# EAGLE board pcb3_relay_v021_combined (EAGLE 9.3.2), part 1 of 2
2022-05-20: PCB made by JLCPCB
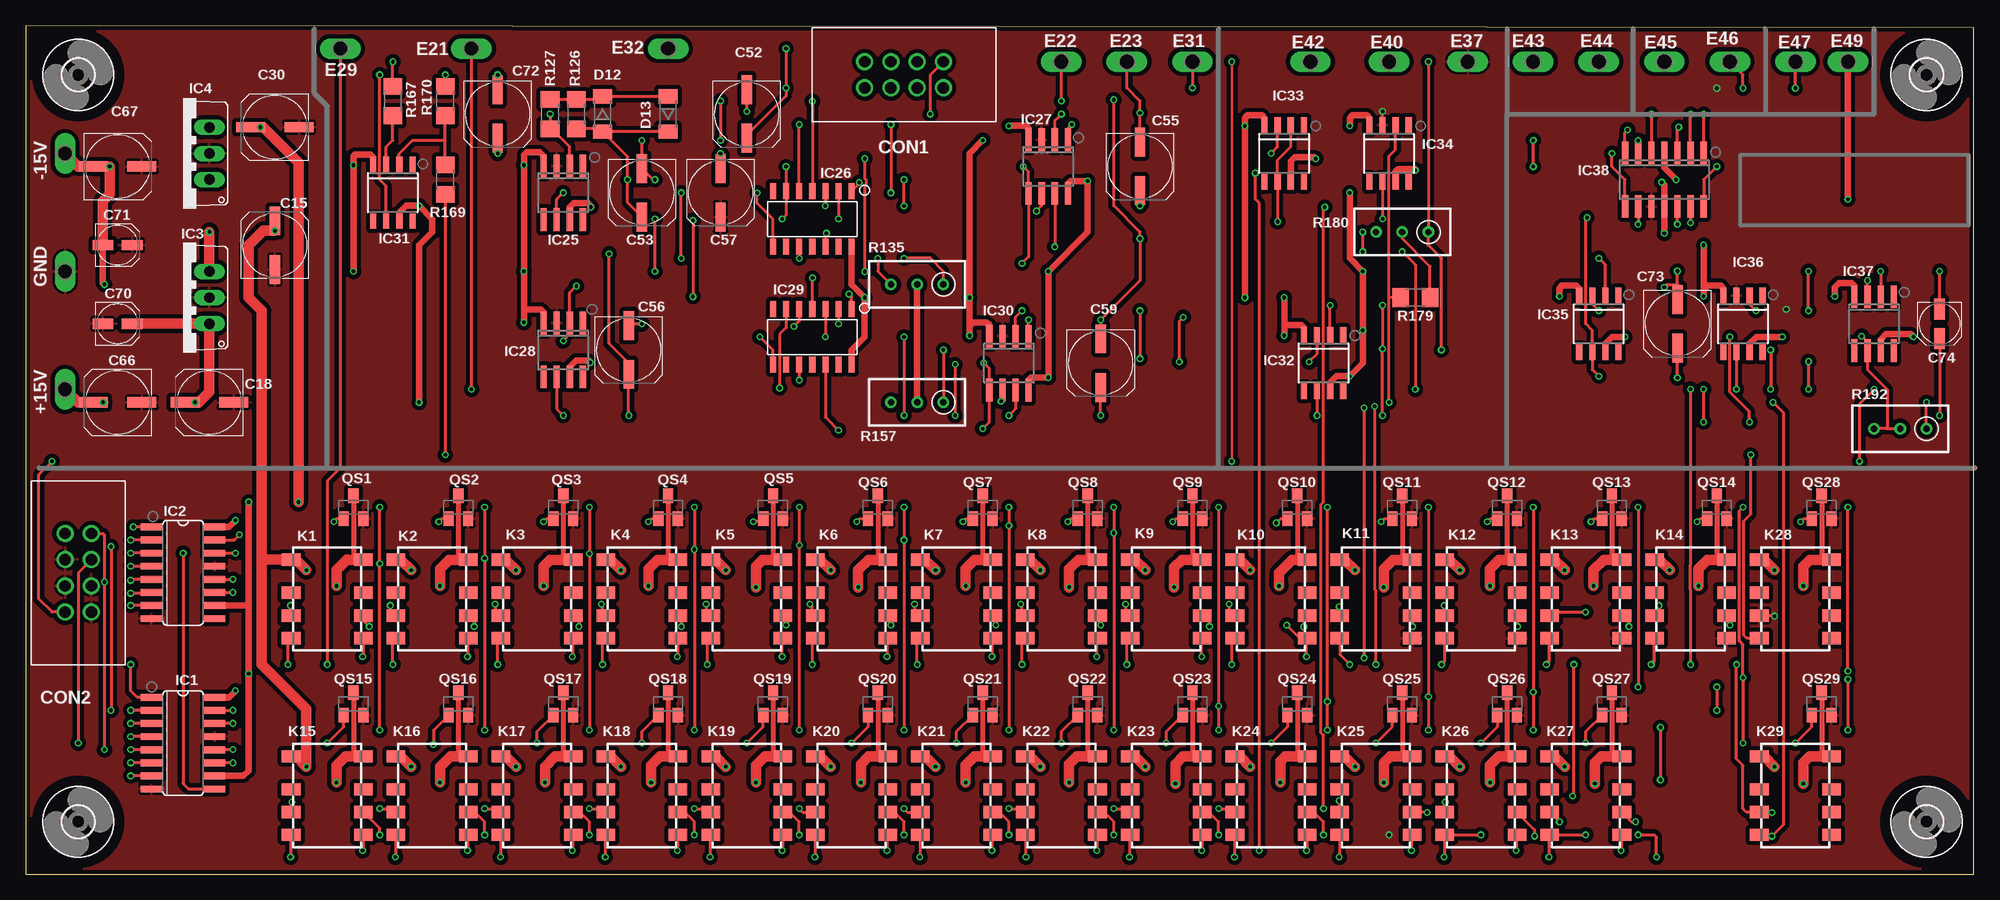
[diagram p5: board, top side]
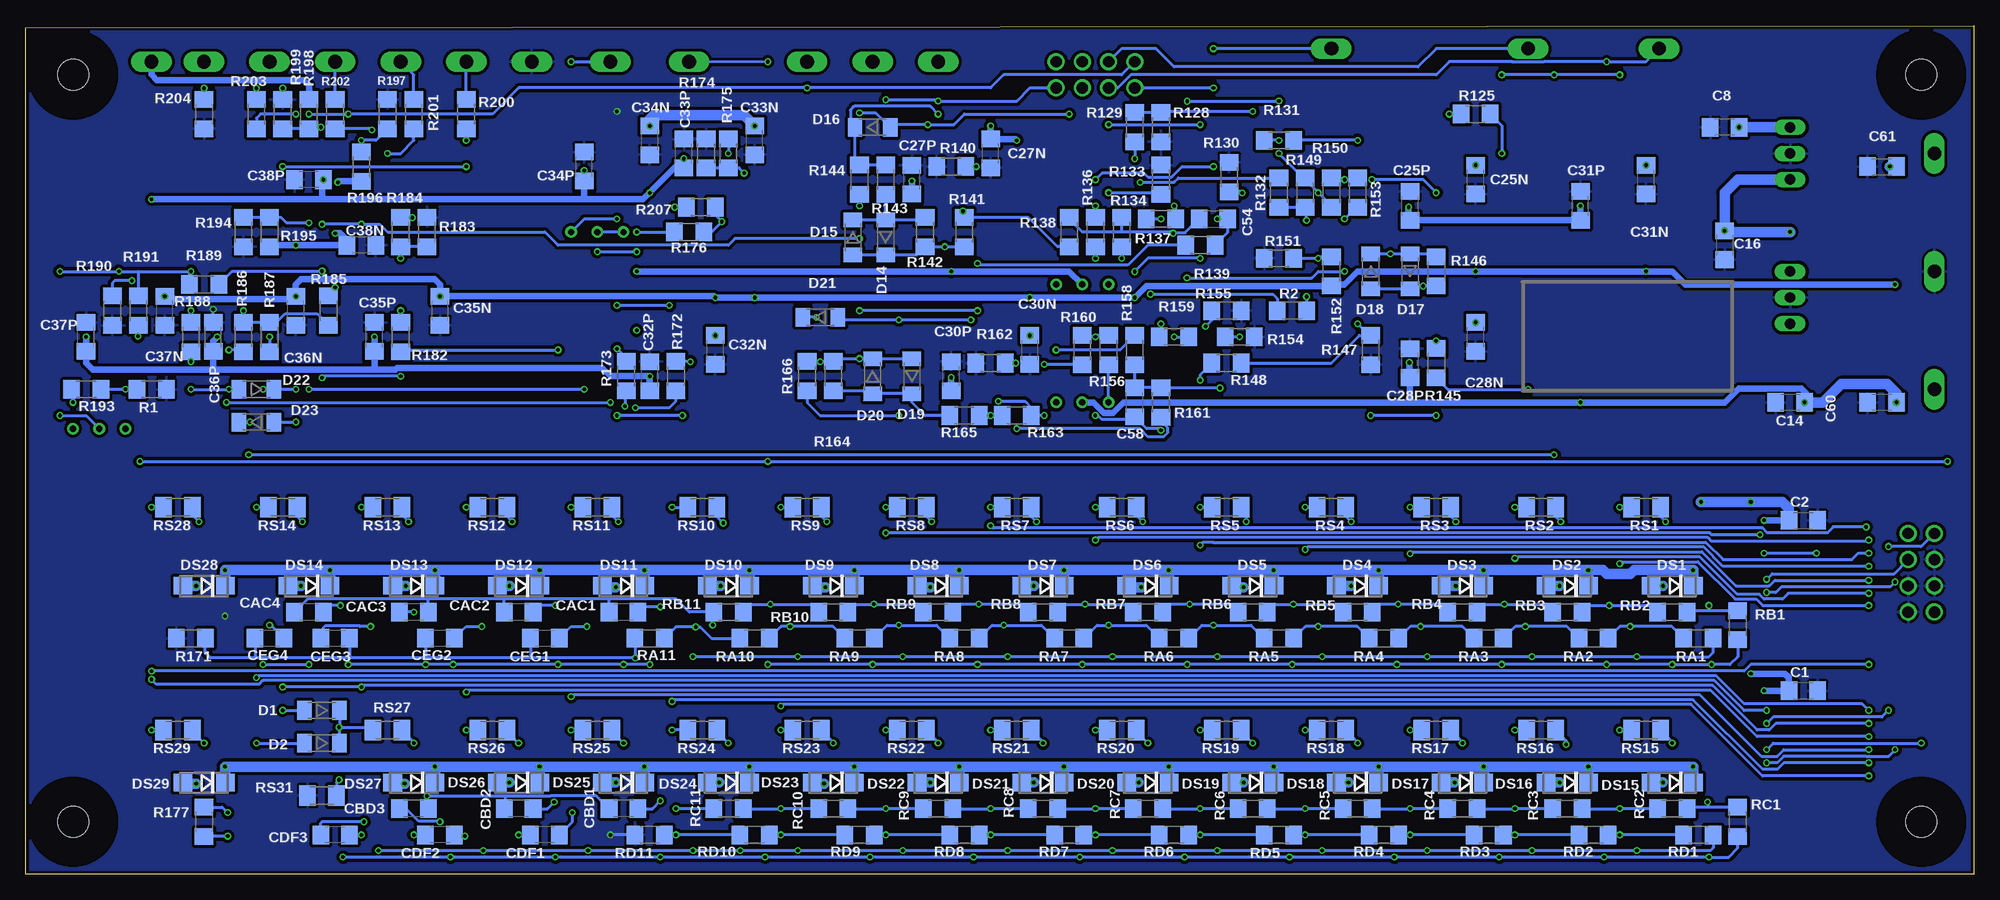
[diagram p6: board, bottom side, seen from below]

Size 188.72 x 82.22 mm. Coordinates in mm from the lower left corner, seen from the top.
Outline: 0,0 188.72,0 188.72,82.04 0,82.22 0,0
Copper layers (1*16): Top 0.035mm / dielectric 1.5mm / Bottom 0.035mm
Design rules "ITEADstudio_DRC for Eagle v6": minimum track width 6mil, minimum drill 12mil, track to track 6mil, track to pad 6mil, pad to pad 6mil, via to via 6mil, smd to smd 0mil, copper to edge 10mil, drill to drill 10mil, minimum pad ring 10mil, minimum via ring 6mil, stop-mask expansion 2mil, vias tented up to drill 100mil, thermal gap 10mil

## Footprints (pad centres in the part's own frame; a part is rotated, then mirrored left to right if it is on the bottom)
P1-13Y = drill 1.321 pad 1.905 long: TP 0,0
C1206 = smd 1.6 x 1.8: 1 -1.4,0; 2 1.4,0
UD-6,3X5,8_NICHICON = smd 2.8 x 1: + 2.35,0; - -2.35,0
UD-4X5,8_NICHICON = smd 2 x 1: + 1.425,0; - -1.425,0
61200821621 = drill 1.1: 1 -2.54,-1.27; 2 -2.54,1.27; 3 0,-1.27; 4 0,1.27; 5 2.54,-1.27; 6 2.54,1.27; 7 5.08,-1.27; 8 5.08,1.27
SOD80 = smd 1.4 x 1.8: 1 -1.7,0; 2 1.7,0
DO214AC = smd 1.8 x 1.7: A 2.05,0; C -2.05,0
SO16 = smd 0.66 x 2.032: 1 -4.445,-3.073; 2 -3.175,-3.073; 3 -1.905,-3.073; 4 -0.635,-3.073; 5 0.635,-3.073; 6 1.905,-3.073; 7 3.175,-3.073; 8 4.445,-3.073; 9 4.445,3.073; 10 3.175,3.073; 11 1.905,3.073; 12 0.635,3.073; 13 -0.635,3.073; 14 -1.905,3.073; 15 -3.175,3.073; 16 -4.445,3.073
TO220V = drill 1.016 long: 1 -2.54,-2.54; 2 0,-2.54; 3 2.54,-2.54
SO08 = smd 0.6 x 2.2: 1 -1.905,-2.6; 2 -0.635,-2.6; 3 0.635,-2.6; 4 1.905,-2.6; 5 1.905,2.6; 6 0.635,2.6; 7 -0.635,2.6; 8 -1.905,2.6
SOIC-14 = smd 0.6 x 1.55: 1 -3.81,-2.7; 2 -2.54,-2.7; 3 -1.27,-2.7; 4 0,-2.7; 5 1.27,-2.7; 6 2.54,-2.7; 7 3.81,-2.7; 8 3.81,2.7; 9 2.54,2.7; 10 1.27,2.7; 11 0,2.7; 12 -1.27,2.7; 13 -2.54,2.7; 14 -3.81,2.7
SOIC8 = smd 0.6 x 1.5: 1 -1.905,-2.75; 2 -0.635,-2.75; 3 0.635,-2.75; 4 1.905,-2.75; 5 1.905,2.75; 6 0.635,2.75; 7 -0.635,2.75; 8 -1.905,2.75
SO14 = smd 0.6 x 2.2: 1 -3.81,-2.6; 2 -2.54,-2.6; 3 -1.27,-2.6; 4 0,-2.6; 5 1.27,-2.6; 6 2.54,-2.6; 7 3.81,-2.6; 8 3.81,2.6; 9 2.54,2.6; 10 1.27,2.6; 11 0,2.6; 12 -1.27,2.6; 13 -2.54,2.6; 14 -3.81,2.6
G6K-2F-Y = smd 1.2 x 1.8: 1 -3.8,-3.5; 2 -0.6,-3.5; 3 1.6,-3.5; 4 3.8,-3.5; 5 3.8,3.5; 6 1.6,3.5; 7 -0.6,3.5; 8 -3.8,3.5
SOT23 = smd 1 x 1.4: 1 -0.95,-1.1; 2 0.95,-1.1; 3 0,1.1
R1206 = smd 1.6 x 1.803: 1 -1.422,0; 2 1.422,0
RTRIM3296W = drill 0.61: 1 0,-2.54; 2 0,0; 3 0,2.54
M1206 = smd 1.6 x 2: 1 -1.4,0; 2 1.4,0
3,0 = hole 3: 0,0

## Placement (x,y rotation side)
+15V  TPPAD1-13Y  [P1-13Y]  3.81,46.99 0 top
-15V  TPPAD1-13Y  [P1-13Y]  3.81,69.85 0 top
C1  100n  [C1206]  16.51,17.78 0 bottom
C2  100n  [C1206]  16.51,34.29 0 bottom
C8  100n  [C1206]  24.13,72.39 180 bottom
C14  100n  [C1206]  17.78,45.72 180 bottom
C15  100u/16V  [UD-6,3X5,8_NICHICON]  24.13,60.96 90 top
C16  100n  [C1206]  24.13,60.96 270 bottom
C18  100u/16V  [UD-6,3X5,8_NICHICON]  17.78,45.72 180 top
C25N  100n  [C1206]  48.26,67.31 90 bottom
C25P  100n  [C1206]  54.61,64.77 90 bottom
C27N  100n  [C1206]  95.25,69.85 90 bottom
C27P  100n  [C1206]  102.87,67.31 90 bottom
C28N  100n  [C1206]  48.26,52.07 90 bottom
C28P  100n  [C1206]  54.61,49.53 90 bottom
C30  100u/16V  [UD-6,3X5,8_NICHICON]  24.13,72.39 180 top
C30N  100n  [C1206]  91.44,50.8 90 bottom
C30P  100n  [C1206]  99.06,48.26 90 bottom
C31N  100n  [C1206]  31.75,67.31 90 bottom
C31P  100n  [C1206]  38.1,64.77 90 bottom
C32N  100n  [C1206]  121.92,50.8 90 bottom
C32P  100n  [C1206]  128.27,48.26 90 bottom
C33N  100n  [C1206]  118.11,71.12 90 bottom
C33P  100n  [C1206]  124.97,69.85 90 bottom
C34N  100n  [C1206]  128.27,71.12 90 bottom
C34P  100n  [C1206]  134.62,68.58 90 bottom
C35N  100n  [C1206]  148.59,54.61 90 bottom
C35P  100n  [C1206]  154.94,52.07 90 bottom
C36N  100n  [C1206]  162.56,54.61 90 bottom
C36P  100n  [C1206]  170.56,52.07 90 bottom
C37N  100n  [C1206]  175.26,54.61 90 bottom
C37P  100n  [C1206]  182.88,52.07 90 bottom
C38N  100n  [C1206]  156.21,60.96 180 bottom
C38P  100n  [C1206]  161.29,67.31 180 bottom
C52  100u/16V  [UD-6,3X5,8_NICHICON]  69.85,73.66 270 top
C53  100u/16V  [UD-6,3X5,8_NICHICON]  59.69,66.04 270 top
C54  0.47uF  [C1206]  73.66,63.5 0 bottom
C55  100u/16V  [UD-6,3X5,8_NICHICON]  107.95,68.58 270 top
C56  100u/16V  [UD-6,3X5,8_NICHICON]  58.42,50.8 270 top
C57  100u/16V  [UD-6,3X5,8_NICHICON]  67.31,66.04 270 top
C58  0.47uF  [C1206]  81.28,45.72 90 bottom
C59  100u/16V  [UD-6,3X5,8_NICHICON]  104.14,49.53 270 top
C60  100n  [C1206]  8.89,45.72 180 bottom
C61  100n  [C1206]  8.89,68.58 0 bottom
C66  100u/16V  [UD-6,3X5,8_NICHICON]  8.89,45.72 180 top
C67  100u/16V  [UD-6,3X5,8_NICHICON]  8.89,68.58 0 top
C70  1u/50V  [UD-4X5,8_NICHICON]  8.89,53.34 0 top
C71  1u/50V  [UD-4X5,8_NICHICON]  8.89,60.96 0 top
C72  100u/16V  [UD-6,3X5,8_NICHICON]  45.72,73.66 270 top
C73  100u/16V  [UD-6,3X5,8_NICHICON]  160.02,53.34 270 top
C74  1u/50V  [UD-4X5,8_NICHICON]  185.42,53.34 270 top
CAC1  100n  [C1206]  130.81,25.4 180 bottom
CAC2  10n  [C1206]  140.97,25.4 180 bottom
CAC3  1n  [C1206]  151.13,25.4 180 bottom
CAC4  100p  [C1206]  161.29,25.4 180 bottom
CBD1  220n  [C1206]  130.81,6.35 180 bottom
CBD2  22n  [C1206]  140.97,6.35 180 bottom
CBD3  2n2  [C1206]  151.13,6.35 180 bottom
CDF1  220n  [C1206]  138.43,3.81 180 bottom
CDF2  22n  [C1206]  148.59,3.81 180 bottom
CDF3  2n2  [C1206]  158.75,3.81 180 bottom
CEG1  68n  [C1206]  138.43,22.86 180 bottom
CEG2  6n8  [C1206]  148.59,22.86 180 bottom
CEG3  680p  [C1206]  158.75,22.86 180 bottom
CEG4  47p  [C1206]  165.1,22.86 180 bottom
CON1  PCB2_IO  [61200821621]  83.82,77.47 0 top
CON2  UC_IO  [61200821621]  5.08,27.94 90 top
D1  1N4148  [SOD80]  160.02,15.88 180 bottom
D2  1N4148  [SOD80]  160.02,12.7 180 bottom
D12  1N4148  [SOD80]  55.88,73.66 270 top
D13  1N4148  [SOD80]  62.23,73.66 90 top
D14  1N4148  [SOD80]  105.41,61.72 90 bottom
D15  1N4148  [SOD80]  108.58,61.72 270 bottom
D16  1N4148  [SOD80]  106.68,72.39 0 bottom
D17  1N4148  [SOD80]  54.61,58.42 90 bottom
D18  1N4148  [SOD80]  58.42,58.42 270 bottom
D19  1N4148  [SOD80]  102.87,48.26 90 bottom
D20  1N4148  [SOD80]  106.68,48.26 270 bottom
D21  1N4148  [SOD80]  111.76,53.98 0 bottom
D22  1N4148  [SOD80]  166.37,46.99 180 bottom
D23  1N4148  [SOD80]  166.37,43.81 0 bottom
DS1  M7  [DO214AC]  29.21,27.94 180 bottom
DS2  M7  [DO214AC]  39.37,27.94 180 bottom
DS3  M7  [DO214AC]  49.53,27.94 180 bottom
DS4  M7  [DO214AC]  59.69,27.94 180 bottom
DS5  M7  [DO214AC]  69.85,27.94 180 bottom
DS6  M7  [DO214AC]  80.01,27.94 180 bottom
DS7  M7  [DO214AC]  90.17,27.94 180 bottom
DS8  M7  [DO214AC]  100.33,27.94 180 bottom
DS9  M7  [DO214AC]  110.49,27.94 180 bottom
DS10  M7  [DO214AC]  120.65,27.94 180 bottom
DS11  M7  [DO214AC]  130.81,27.94 180 bottom
DS12  M7  [DO214AC]  140.97,27.94 180 bottom
DS13  M7  [DO214AC]  151.13,27.94 180 bottom
DS14  M7  [DO214AC]  161.29,27.94 180 bottom
DS15  M7  [DO214AC]  29.21,8.89 180 bottom
DS16  M7  [DO214AC]  39.37,8.89 180 bottom
DS17  M7  [DO214AC]  49.53,8.89 180 bottom
DS18  M7  [DO214AC]  59.69,8.89 180 bottom
DS19  M7  [DO214AC]  69.85,8.89 180 bottom
DS20  M7  [DO214AC]  80.01,8.89 180 bottom
DS21  M7  [DO214AC]  90.17,8.89 180 bottom
DS22  M7  [DO214AC]  100.33,8.89 180 bottom
DS23  M7  [DO214AC]  110.49,8.89 180 bottom
DS24  M7  [DO214AC]  120.65,8.89 180 bottom
DS25  M7  [DO214AC]  130.81,8.89 180 bottom
DS26  M7  [DO214AC]  140.97,8.89 180 bottom
DS27  M7  [DO214AC]  151.13,8.89 180 bottom
DS28  M7  [DO214AC]  171.45,27.94 180 bottom
DS29  M7  [DO214AC]  171.45,8.89 180 bottom
E21  TPPAD1-13Y  [P1-13Y]  43.18,80.01 90 top
E22  TPPAD1-13Y  [P1-13Y]  100.33,78.74 90 top
E23  TPPAD1-13Y  [P1-13Y]  106.68,78.74 90 top
E29  TPPAD1-13Y  [P1-13Y]  30.48,80.01 270 top
E31  TPPAD1-13Y  [P1-13Y]  113.03,78.74 90 top
E32  TPPAD1-13Y  [P1-13Y]  62.23,80.01 90 top
E37  TPPAD1-13Y  [P1-13Y]  139.7,78.74 90 top
E40  TPPAD1-13Y  [P1-13Y]  132.08,78.74 90 top
E42  TPPAD1-13Y  [P1-13Y]  124.46,78.74 90 top
E43  TPPAD1-13Y  [P1-13Y]  146.05,78.74 90 top
E44  TPPAD1-13Y  [P1-13Y]  152.4,78.74 90 top
E45  TPPAD1-13Y  [P1-13Y]  158.75,78.74 90 top
E46  TPPAD1-13Y  [P1-13Y]  165.1,78.74 90 top
E47  TPPAD1-13Y  [P1-13Y]  171.45,78.74 90 top
E49  TPPAD1-13Y  [P1-13Y]  176.53,78.74 90 top
GND  TPPAD1-13Y  [P1-13Y]  3.81,58.42 0 top
IC1  74HC595D  [SO16]  15.24,12.7 270 top
IC2  74HC595D  [SO16]  15.24,29.21 270 top
IC3  7812TV  [TO220V]  15.24,55.88 90 top
IC4  7805TV  [TO220V]  15.24,69.85 90 top
IC25  LM318D  [SO08]  52.07,66.04 180 top
IC26  MC1496D  [SOIC-14]  76.2,63.5 180 top
IC27  LM1458D  [SO08]  99.06,68.58 180 top
IC28  LM318D  [SO08]  52.07,50.8 180 top
IC29  MC1496D  [SOIC-14]  76.2,52.07 180 top
IC30  LM1458D  [SO08]  95.25,49.53 180 top
IC31  LM318D  [SOIC8]  35.56,66.04 180 top
IC32  LM318D  [SOIC8]  125.73,49.53 180 top
IC33  LM318D  [SOIC8]  121.92,69.85 180 top
IC34  LM318D  [SOIC8]  132.08,69.85 180 top
IC35  LM318D  [SOIC8]  152.4,53.34 180 top
IC36  LM318D  [SOIC8]  166.37,53.34 180 top
IC37  LM741D  [SO08]  179.07,53.34 180 top
IC38  LM324D  [SO14]  158.75,67.31 180 top
K1  G6K-2F-Y  [G6K-2F-Y]  29.21,26.67 270 top
K2  G6K-2F-Y  [G6K-2F-Y]  39.37,26.67 270 top
K3  G6K-2F-Y  [G6K-2F-Y]  49.53,26.67 270 top
K4  G6K-2F-Y  [G6K-2F-Y]  59.69,26.67 270 top
K5  G6K-2F-Y  [G6K-2F-Y]  69.85,26.67 270 top
K6  G6K-2F-Y  [G6K-2F-Y]  80.01,26.67 270 top
K7  G6K-2F-Y  [G6K-2F-Y]  90.17,26.67 270 top
K8  G6K-2F-Y  [G6K-2F-Y]  100.33,26.67 270 top
K9  G6K-2F-Y  [G6K-2F-Y]  110.49,26.67 270 top
K10  G6K-2F-Y  [G6K-2F-Y]  120.65,26.67 270 top
K11  G6K-2F-Y  [G6K-2F-Y]  130.81,26.67 270 top
K12  G6K-2F-Y  [G6K-2F-Y]  140.97,26.67 270 top
K13  G6K-2F-Y  [G6K-2F-Y]  151.13,26.67 270 top
K14  G6K-2F-Y  [G6K-2F-Y]  161.29,26.67 270 top
K15  G6K-2F-Y  [G6K-2F-Y]  29.21,7.62 270 top
K16  G6K-2F-Y  [G6K-2F-Y]  39.37,7.62 270 top
K17  G6K-2F-Y  [G6K-2F-Y]  49.53,7.62 270 top
K18  G6K-2F-Y  [G6K-2F-Y]  59.69,7.62 270 top
K19  G6K-2F-Y  [G6K-2F-Y]  69.85,7.62 270 top
K20  G6K-2F-Y  [G6K-2F-Y]  80.01,7.62 270 top
K21  G6K-2F-Y  [G6K-2F-Y]  90.17,7.62 270 top
K22  G6K-2F-Y  [G6K-2F-Y]  100.33,7.62 270 top
K23  G6K-2F-Y  [G6K-2F-Y]  110.49,7.62 270 top
K24  G6K-2F-Y  [G6K-2F-Y]  120.65,7.62 270 top
K25  G6K-2F-Y  [G6K-2F-Y]  130.81,7.62 270 top
K26  G6K-2F-Y  [G6K-2F-Y]  140.97,7.62 270 top
K27  G6K-2F-Y  [G6K-2F-Y]  151.13,7.62 270 top
K28  G6K-2F-Y  [G6K-2F-Y]  171.45,26.67 270 top
K29  G6K-2F-Y  [G6K-2F-Y]  171.45,7.62 270 top
QS1  SS8050  [SOT23]  31.75,35.56 0 top
QS2  SS8050  [SOT23]  41.91,35.56 0 top
QS3  SS8050  [SOT23]  52.07,35.56 0 top
QS4  SS8050  [SOT23]  62.23,35.56 0 top
QS5  SS8050  [SOT23]  72.39,35.56 0 top
QS6  SS8050  [SOT23]  82.55,35.56 0 top
QS7  SS8050  [SOT23]  92.71,35.56 0 top
QS8  SS8050  [SOT23]  102.87,35.56 0 top
QS9  SS8050  [SOT23]  113.03,35.56 0 top
QS10  SS8050  [SOT23]  123.19,35.56 0 top
QS11  SS8050  [SOT23]  133.35,35.56 0 top
QS12  SS8050  [SOT23]  143.51,35.56 0 top
QS13  SS8050  [SOT23]  153.67,35.56 0 top
QS14  SS8050  [SOT23]  163.83,35.56 0 top
QS15  SS8050  [SOT23]  31.75,16.51 0 top
QS16  SS8050  [SOT23]  41.91,16.51 0 top
QS17  SS8050  [SOT23]  52.07,16.51 0 top
QS18  SS8050  [SOT23]  62.23,16.51 0 top
QS19  SS8050  [SOT23]  72.39,16.51 0 top
QS20  SS8050  [SOT23]  82.55,16.51 0 top
QS21  SS8050  [SOT23]  92.71,16.51 0 top
QS22  SS8050  [SOT23]  102.87,16.51 0 top
QS23  SS8050  [SOT23]  113.03,16.51 0 top
QS24  SS8050  [SOT23]  123.19,16.51 0 top
QS25  SS8050  [SOT23]  133.35,16.51 0 top
QS26  SS8050  [SOT23]  143.51,16.51 0 top
QS27  SS8050  [SOT23]  153.67,16.51 0 top
QS28  SS8050  [SOT23]  173.99,35.56 0 top
QS29  SS8050  [SOT23]  173.99,16.51 0 top
R1  3K3  [R1206]  176.53,46.99 180 bottom
R2  100  [R1206]  66.04,54.61 180 bottom
R125  4K7  [R1206]  48.26,73.66 0 bottom
R126  22k  [R1206]  53.34,73.66 270 top
R127  2K7  [R1206]  50.8,73.66 90 top
R128  1K  [R1206]  78.74,72.39 270 bottom
R129  100  [R1206]  81.28,72.39 90 bottom
R130  100  [R1206]  72.14,67.56 90 bottom
R131  100  [R1206]  67.31,71.12 0 bottom
R132  100  [R1206]  67.31,66.04 270 bottom
R133  22k  [R1206]  78.74,67.31 90 bottom
R134  10k  [R1206]  82.55,62.23 90 bottom
R135  1k  [RTRIM3296W]  86.36,57.15 90 top
R136  10k  [R1206]  85.09,62.23 270 bottom
R137  1K5  [R1206]  78.74,63.5 0 bottom
R138  22k  [R1206]  87.63,62.23 90 bottom
R139  22k  [R1206]  74.93,60.96 180 bottom
R140  6K8  [R1206]  99.06,68.58 180 bottom
R141  6K8  [R1206]  97.79,62.23 90 bottom
R142  100k  [R1206]  101.6,62.23 270 bottom
R143  10k  [R1206]  105.41,67.31 270 bottom
R144  68  [R1206]  107.95,67.31 90 bottom
R145  10k  [R1206]  52.07,49.53 270 bottom
R146  100k  [R1206]  52.07,58.42 90 bottom
R147  10k  [R1206]  58.42,50.8 270 bottom
R148  100  [R1206]  72.39,49.53 0 bottom
R149  1K  [R1206]  64.77,66.04 270 bottom
R150  1K  [R1206]  62.23,66.04 90 bottom
R151  4K7  [R1206]  67.31,59.69 0 bottom
R152  4K7  [R1206]  62.23,58.42 90 bottom
R153  100  [R1206]  59.69,66.04 270 bottom
R154  100  [R1206]  71.12,52.07 0 bottom
R155  22k  [R1206]  72.39,54.61 0 bottom
R156  10k  [R1206]  83.82,50.8 90 bottom
R157  1k  [RTRIM3296W]  86.36,45.72 90 top
R158  10k  [R1206]  81.28,50.8 90 bottom
R159  1K5  [R1206]  77.47,52.07 0 bottom
R160  22k  [R1206]  86.36,50.8 90 bottom
R161  22k  [R1206]  78.74,45.72 270 bottom
R162  6K8  [R1206]  95.25,49.53 180 bottom
R163  6K8  [R1206]  92.71,44.45 0 bottom
R164  100k  [R1206]  110.49,48.26 270 bottom
R165  10k  [R1206]  97.79,44.45 0 bottom
R166  68  [R1206]  113.03,48.26 90 bottom
R167  100  [R1206]  35.56,74.93 270 top
R169  390  [R1206]  40.64,67.31 270 top
R170  3K3  [R1206]  40.64,74.93 270 top
R171  100k  [R1206]  172.72,22.86 0 bottom
R172  100  [R1206]  125.73,48.26 90 bottom
R173  100  [R1206]  130.56,48.26 270 bottom
R174  100k  [R1206]  122.81,69.85 270 bottom
R175  100  [R1206]  120.65,69.85 90 bottom
R176  1K  [R1206]  124.46,62.23 180 bottom
R177  9k09  [R1206]  171.45,5.08 270 bottom
R179  3K  [R1206]  134.62,55.88 0 top
R180  2K  [RTRIM3296W]  133.35,62.23 90 top
R182  100  [R1206]  152.4,52.07 90 bottom
R183  1K  [R1206]  149.86,62.23 90 bottom
R184  9K1  [R1206]  152.4,62.23 270 bottom
R185  1K  [R1206]  159.38,54.61 90 bottom
R186  1K  [R1206]  167.64,52.07 270 bottom
R187  1K  [R1206]  165.1,52.07 90 bottom
R188  10k  [R1206]  172.72,52.07 90 bottom
R189  20k  [R1206]  171.45,57.15 0 bottom
R190  6K8  [R1206]  180.34,54.61 90 bottom
R191  270k  [R1206]  177.8,54.61 270 bottom
R192  5k  [RTRIM3296W]  181.61,43.18 90 top
R193  4K7  [R1206]  182.88,46.99 180 bottom
R194  39k  [R1206]  167.64,62.23 90 bottom
R195  10k  [R1206]  165.1,62.23 90 bottom
R196  33k  [R1206]  156.21,68.58 90 bottom
R197  10k  [R1206]  153.67,73.66 270 bottom
R198  33k  [R1206]  161.29,73.66 270 bottom
R199  10k  [R1206]  163.83,73.66 270 bottom
R200  2K7  [R1206]  146.05,73.66 90 bottom
R201  2K7  [R1206]  151.13,73.66 90 bottom
R202  2K7  [R1206]  158.75,73.66 90 bottom
R203  2K7  [R1206]  166.37,73.66 90 bottom
R204  1K5  [R1206]  171.45,73.66 90 bottom
R207  100  [R1206]  123.32,64.64 0 bottom
RA1  1K5  [R1206]  26.67,22.86 180 bottom
RA2  1K  [R1206]  36.83,22.86 180 bottom
RA3  1K3  [R1206]  46.99,22.86 180 bottom
RA4  750  [R1206]  57.15,22.86 180 bottom
RA5  680  [R1206]  67.31,22.86 180 bottom
RA6  430  [R1206]  77.47,22.86 180 bottom
RA7  360  [R1206]  87.63,22.86 180 bottom
RA8  330  [R1206]  97.79,22.86 180 bottom
RA9  220  [R1206]  107.95,22.86 180 bottom
RA10  180  [R1206]  118.11,22.86 180 bottom
RA11  750  [R1206]  128.27,22.86 180 bottom
RB1  1K5  [R1206]  22.86,24.13 90 bottom
RB2  1K  [R1206]  29.21,25.4 180 bottom
RB3  1K3  [R1206]  39.37,25.4 180 bottom
RB4  750  [R1206]  49.53,25.4 180 bottom
RB5  680  [R1206]  59.69,25.4 180 bottom
RB6  430  [R1206]  69.85,25.4 180 bottom
RB7  360  [R1206]  80.01,25.4 180 bottom
RB8  330  [R1206]  90.17,25.4 180 bottom
RB9  220  [R1206]  100.33,25.4 180 bottom
RB10  180  [R1206]  110.49,25.4 180 bottom
RB11  750  [R1206]  120.65,25.4 180 bottom
RC1  3K6  [R1206]  22.86,5.08 90 bottom
RC2  2K4  [R1206]  29.21,6.35 180 bottom
RC3  3K  [R1206]  39.37,6.35 180 bottom
RC4  1K8  [R1206]  49.53,6.35 180 bottom
RC5  1K6  [R1206]  59.69,6.35 180 bottom
RC6  1K  [R1206]  69.85,6.35 180 bottom
RC7  910  [R1206]  80.01,6.35 180 bottom
RC8  820  [R1206]  90.17,6.35 180 bottom
RC9  510  [R1206]  100.33,6.35 180 bottom
RC10  470  [R1206]  110.49,6.35 180 bottom
RC11  1K8  [R1206]  120.65,6.35 180 bottom
RD1  9K1  [R1206]  26.67,3.81 180 bottom
RD2  6K8  [R1206]  36.83,3.81 180 bottom
RD3  7K5  [R1206]  46.99,3.81 180 bottom
RD4  4K7  [R1206]  57.15,3.81 180 bottom
RD5  4K3  [R1206]  67.31,3.81 180 bottom
RD6  2K7  [R1206]  77.47,3.81 180 bottom
RD7  2K4  [R1206]  87.63,3.81 180 bottom
RD8  2K2  [R1206]  97.79,3.81 180 bottom
RD9  1K3  [R1206]  107.95,3.81 180 bottom
RD10  1K2  [R1206]  118.11,3.81 180 bottom
RD11  4K7  [R1206]  128.27,3.81 180 bottom
RS1  4k7  [M1206]  31.75,35.56 180 bottom
RS2  4k7  [M1206]  41.91,35.56 180 bottom
RS3  4k7  [M1206]  52.07,35.56 180 bottom
RS4  4k7  [M1206]  62.23,35.56 180 bottom
RS5  4k7  [M1206]  72.39,35.56 180 bottom
RS6  4k7  [M1206]  82.55,35.56 180 bottom
RS7  4k7  [M1206]  92.71,35.56 180 bottom
RS8  4k7  [M1206]  102.87,35.56 180 bottom
RS9  4k7  [M1206]  113.03,35.56 180 bottom
RS10  4k7  [M1206]  123.19,35.56 180 bottom
RS11  4k7  [M1206]  133.35,35.56 180 bottom
RS12  4k7  [M1206]  143.51,35.56 180 bottom
RS13  4k7  [M1206]  153.67,35.56 180 bottom
RS14  4k7  [M1206]  163.83,35.56 180 bottom
RS15  4k7  [M1206]  31.75,13.97 180 bottom
RS16  4k7  [M1206]  41.91,13.97 180 bottom
RS17  4k7  [M1206]  52.07,13.97 180 bottom
RS18  4k7  [M1206]  62.23,13.97 180 bottom
RS19  4k7  [M1206]  72.39,13.97 180 bottom
RS20  4k7  [M1206]  82.55,13.97 180 bottom
RS21  4k7  [M1206]  92.71,13.97 180 bottom
RS22  4k7  [M1206]  102.87,13.97 180 bottom
RS23  4k7  [M1206]  113.03,13.97 180 bottom
RS24  4k7  [M1206]  123.19,13.97 180 bottom
RS25  4k7  [M1206]  133.35,13.97 180 bottom
RS26  4k7  [M1206]  143.51,13.97 180 bottom
RS27  4k7  [M1206]  153.67,13.97 180 bottom
RS28  4k7  [M1206]  173.99,35.56 180 bottom
RS29  4k7  [M1206]  173.99,13.97 180 bottom
RS31  4k7  [M1206]  160.02,7.62 180 bottom
U$1  [3,0]  5.08,5.08 0 top
U$2  [3,0]  5.08,77.47 0 top
U$3  [3,0]  184.15,77.47 0 top
U$4  [3,0]  184.15,5.08 0 top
